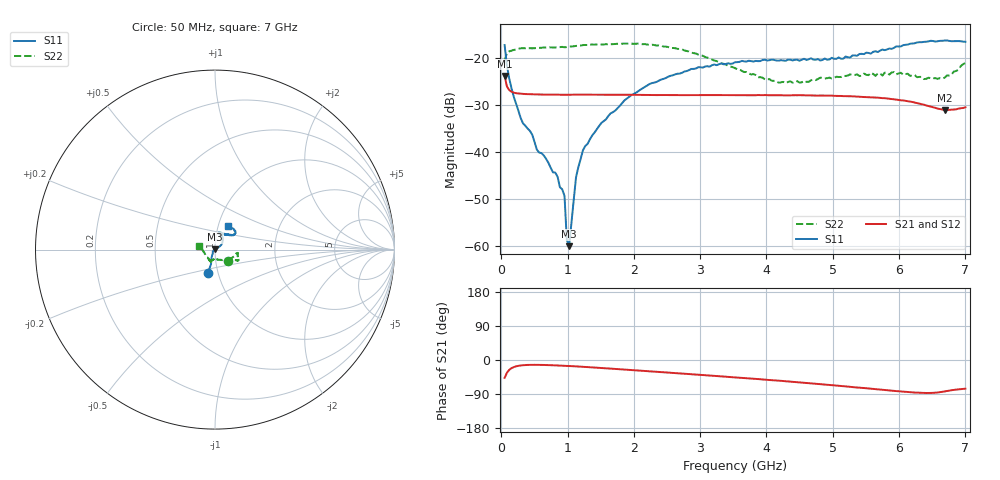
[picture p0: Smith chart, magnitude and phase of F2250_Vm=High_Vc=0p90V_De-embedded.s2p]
! Integrated Device Technology
! Corporate Headquarters
! 6024 Silver Creek Valley Road
! San Jose, CA 95138  USA
! Phone:  1-408-284-8200
! Toll Free:  1-800-223-1366
! Webpage:  http://www.idt.com/
! Timing and RF Division
! 515 Groton Road, Suite 102
! Westford, MA 01886-6024
! Device:  F2250
! Description: Voltage Variable RF Attenuator
! Frequency:  50.0 -  6000.00 MHz
! Package:  3x3 mm Thin QFN Plastic Package: 16 pin
! Ports:  2 RF, 3 DC
!  Pin  1  = GND
!  Pin  2  = NC
!  Pin  3  = RF1  = Port 1
!  Pin  4  = NC
!  Pin  5  = GND
!  Pin  6  = GND
!  Pin  7  = GND
!  Pin  8  = GND
!  Pin  9  = NC
!  Pin 10  = RF2  = Port 2
!  Pin 11  = NC
!  Pin 12  = GND
!  Pin 13  = GND
!  Pin 14  = VCNTRL
!  Pin 15  = VDD
!  Pin 16  = VMODE
! Vcntrl:  0.900 Volts
! Vmode:  +3.300 Volts
! Vdd:  +3.30  Volts
! Current:  1.316 mA
! Data:  The device was measured on a the F2250 evaluation board which has
!  individual transmission lines to the RF pins.  Data was collected
!  using a calibrated network analyzer.  The evaluation board was
!  de-embedded using a TRL calibration technique.
!  The reference plane is the edge of the package pin.
! Misc:  SN 10
!  Action Tracker AT0258
! Date Measured:  2014-11-26
! Date:  2015-10-15  MJV
! Note:
!  Integrated Device Technology supplies this data as a sample of measured
!  data at the package pin for this product.  Your particular data for this
!  product may vary.
!  Data was taken at 25 degrees C.
!  Integrated Device Technology reserves the right to change this data at anytime.
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# GHz S dB R 50
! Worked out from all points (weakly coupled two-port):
!   201 points, 50 MHz to 7 GHz, reference 50 ohm
!   highest |S21| = -23.72 dB at 50 MHz (marker M1); lowest = -31.0 dB at 6.687 GHz (marker M2)
!   lowest |S11| = -60.0 dB at 1.023 GHz (marker M3), VSWR 1.00, Z = 50 + j0.0948 ohm
!   |S11| at or under -10 dB: start of sweep to end of sweep
!   |S22| runs from -25.3 to -16.9 dB; largest |S21 - S12| = 0.00021
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0.05  -17.17 -106.9  -23.72 -47.1  -23.72 -47.1  -20.51 -40.3
0.08475  -21.50 -105.3  -25.97 -33.7  -25.97 -33.6  -18.85 -18.4
0.1195  -24.28 -109.3  -26.76 -26.0  -26.75 -26.0  -18.52 -12.2
0.29325  -32.73 -121.3  -27.51 -14.4  -27.52 -14.4  -17.86 -9.0
0.467  -36.26 -138.8  -27.66 -12.7  -27.64 -12.7  -17.87 -9.0
0.5365  -39.42 -145.5  -27.68 -12.8  -27.67 -12.8  -17.80 -10.2
0.8145  -44.31 172.4  -27.71 -14.2  -27.71 -14.2  -17.69 -14.2
0.9535  -49.26 178.9  -27.74 -15.2  -27.74 -15.3  -17.65 -16.4
0.98825  -58.61 176.5  -27.75 -15.5  -27.75 -15.5  -17.60 -16.8
1.023  -59.96 70.4  -27.75 -15.8  -27.75 -15.8  -17.51 -16.9
1.12725  -45.28 31.3  -27.72 -16.8  -27.73 -16.8  -17.35 -18.2
1.2315  -39.55 27.2  -27.70 -17.9  -27.71 -17.9  -17.18 -19.9
1.5095  -33.74 33.5  -27.73 -21.2  -27.74 -21.2  -17.07 -21.7
1.857  -28.95 35.2  -27.77 -25.2  -27.76 -25.2  -16.86 -24.0
2.37825  -24.73 44.1  -27.81 -31.5  -27.79 -31.5  -17.23 -26.5
2.969  -21.90 58.1  -27.83 -38.7  -27.82 -38.7  -19.20 -30.8
3.525  -20.82 70.5  -27.87 -45.8  -27.85 -45.9  -22.09 -47.6
4.18525  -20.48 76.6  -27.85 -54.5  -27.86 -54.5  -25.20 -79.0
4.7065  -20.27 71.3  -27.89 -62.2  -27.90 -62.2  -24.56 -102.1
5.85325  -17.91 39.9  -28.60 -80.3  -28.61 -80.4  -23.45 -111.4
6.68725  -16.21 47.3  -31.01 -83.0  -31.03 -83.1  -24.12 -166.5
7  -16.47 61.9  -30.42 -75.6  -30.44 -75.6  -20.99 167.6
